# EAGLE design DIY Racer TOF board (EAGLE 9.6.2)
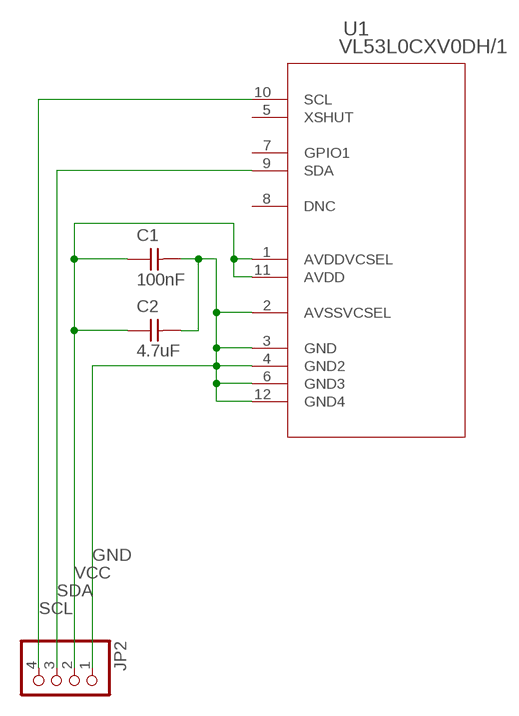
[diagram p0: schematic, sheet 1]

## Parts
C1  100nF  CAP_UNPOLARIZED  [C1206]
C2  4.7uF  CAP_UNPOLARIZED  [C1206]
JP2  PINHD-1X04_2.54-SMD  [1X04SMD]
U1  VL53L0CXV0DH/1  [LGA12_STM]

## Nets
GND: C1.2 C2.2 JP2.1 U1.2(AVSSVCSEL) U1.3(GND) U1.4(GND2) U1.6(GND3) U1.12(GND4)
SCL: JP2.4 U1.10(SCL)
SDA: JP2.3 U1.9(SDA)
VCC: C1.1 C2.1 JP2.2 U1.1(AVDDVCSEL) U1.11(AVDD)
Unconnected: U1.5(XSHUT) U1.7(GPIO1) U1.8(DNC)

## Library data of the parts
C1 C2 = fab:CAP_UNPOLARIZED
JP2 = pinhead-2:PINHD-1X04: PIN HEADER
U1 = VL53L0CXV0DH1:VL53L0CXV0DH/1; BUILT_BY: EMA_Jessica; COPYRIGHT: Copyright (C) 2018 Accelerated Designs. All rights reserved; MANUFACTURER_PART_NUMBER: VL53L0CXV0DH/1; SOURCELIBRARY: Update_to_database_2020-12-04; VENDOR: STMicroelectronics

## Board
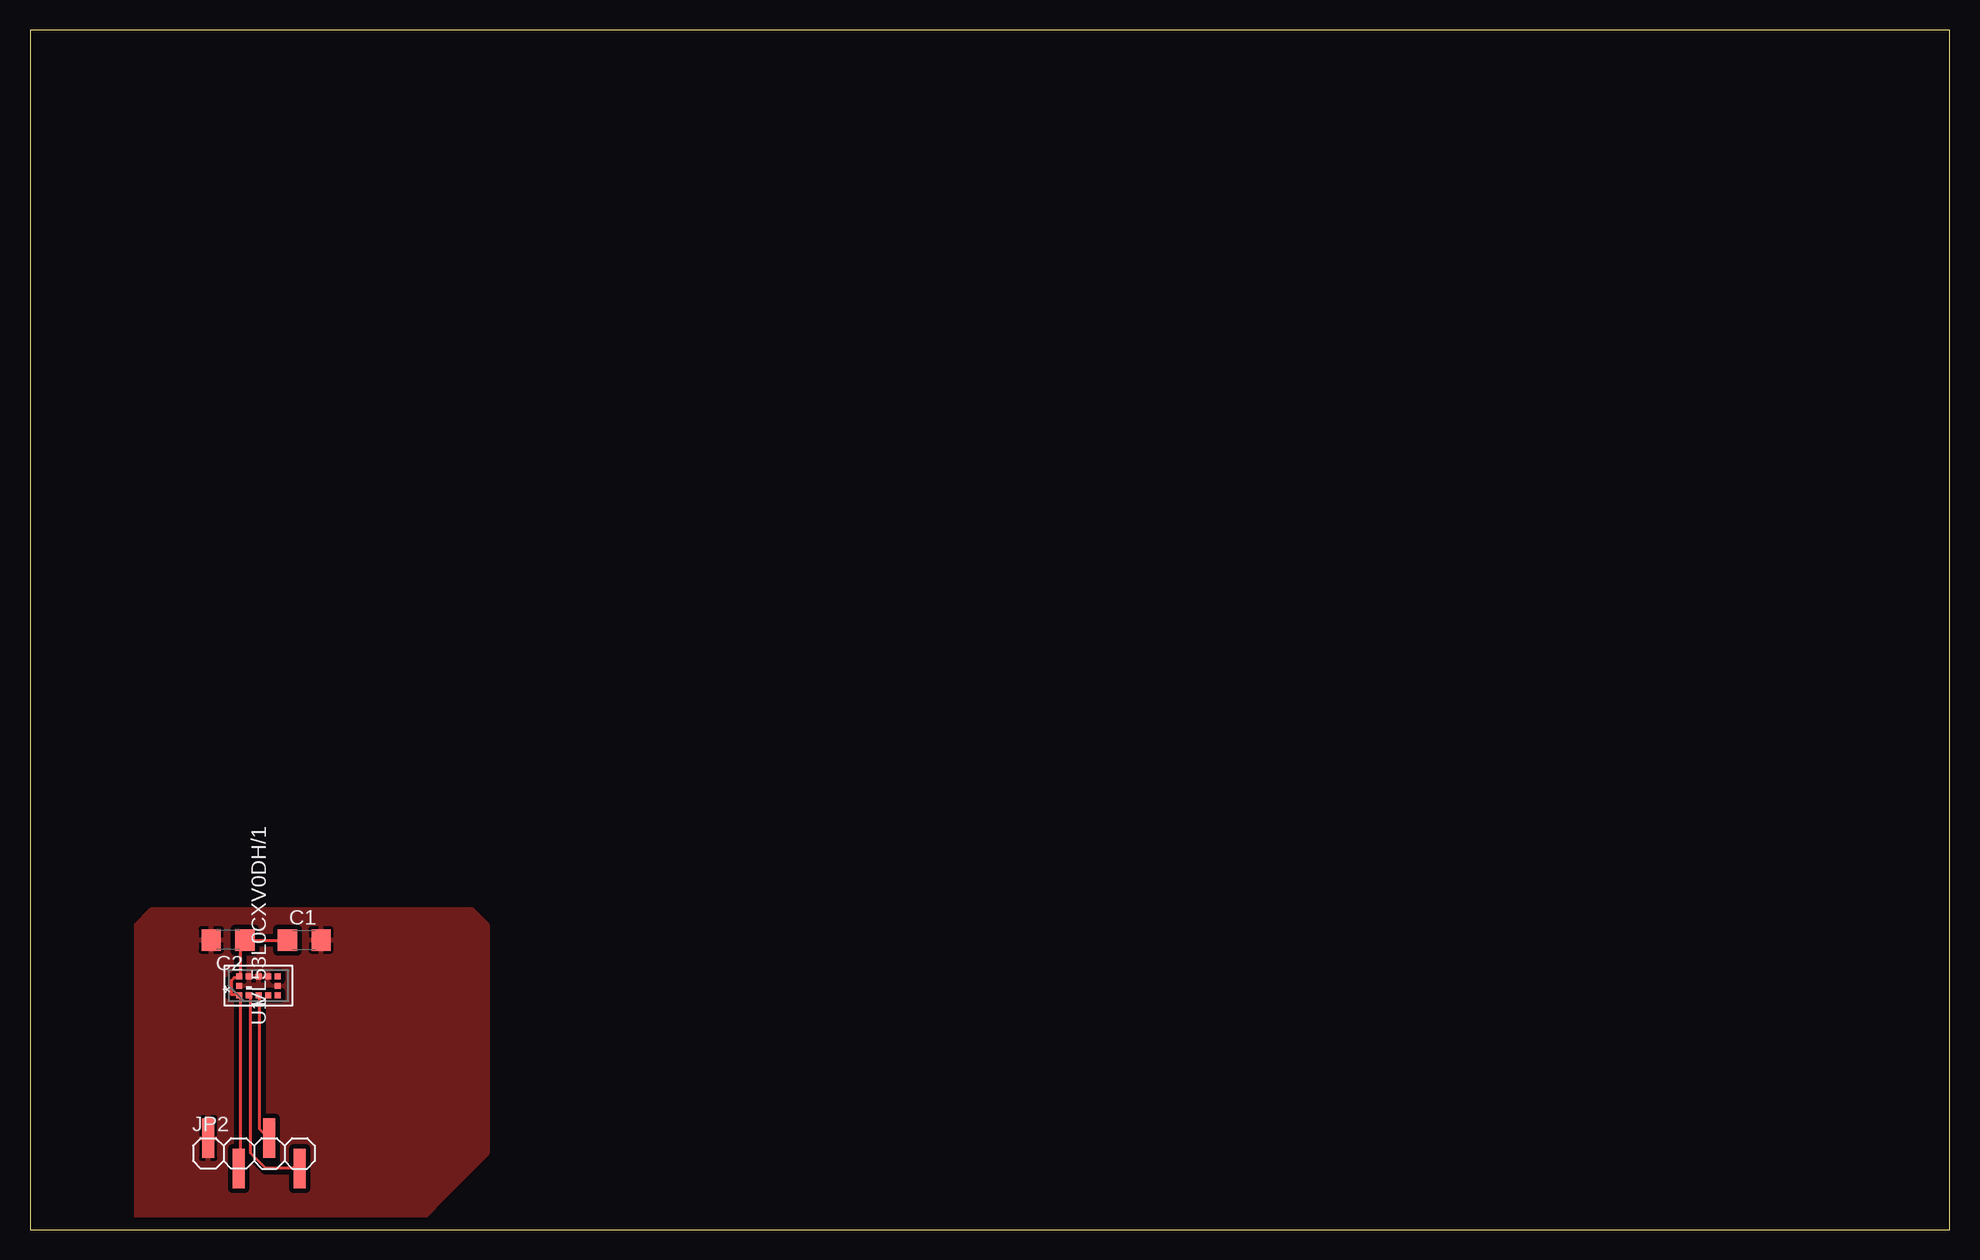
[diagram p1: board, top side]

Size 160 x 100 mm. Coordinates in mm from the lower left corner, seen from the top.
Outline: 0,0 160,0 160,100 0,100 0,0
Copper layers (1*16): Top 0.035mm / dielectric 1.5mm / Bottom 0.035mm
Design rules "default *": minimum track width 0.25mm, minimum drill 0.35mm, track to track 0.4mm, track to pad 0.25mm, pad to pad 0.25mm, via to via 0.4mm, smd to smd 0.25mm, copper to edge 40mil, drill to drill 6mil, minimum pad ring 10mil, minimum via ring 8mil, stop-mask expansion 4mil, vias tented up to drill 0mil, thermal gap 10mil

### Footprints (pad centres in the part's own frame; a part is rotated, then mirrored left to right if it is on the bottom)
C1206 = smd 1.6 x 1.8: 1 -1.4,0; 2 1.4,0
1X04SMD = smd 1.016 x 3.302: 1 -1.27,1.27; 2 1.27,-1.27; 3 3.81,1.27; 4 6.35,-1.27
LGA12_STM = smd 0.508 x 0.508: 1 0.8,1.6; 2 0.8,0.8; 3 0.8,0; 4 0.8,-0.8; 5 0.8,-1.6; 6 0,-1.6; 7 -0.8,-1.6; 8 -0.8,-0.8; 9 -0.8,0; 10 -0.8,0.8; 11 -0.8,1.6; 12 0,1.6

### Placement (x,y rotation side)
C1  22.86,24.13 0 top
C2  16.51,24.13 180 top
JP2  16.13,6.35 0 top
U1  19.05,20.32 90 top

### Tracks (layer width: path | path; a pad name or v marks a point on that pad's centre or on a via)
GND
  pour Top: 10.16,26.67 36.83,26.67 38.1,25.4 38.1,6.35 35.56,3.81 31.75,0 26.67,0 8.89,0 8.89,25.4
SCL
  Top 0.25: U1.10 18.25,19.5 18.38,19.38 18.38,6.38 19.62,5.12 22.38,5.12 JP2.4
SDA
  Top 0.25: U1.9 19.12,19.5 19.12,8.38 19.88,7.62 JP2.3
VCC
  Top 0.25: C1.1 21.38,24.12 18,24.12 C2.1 17.88,24.12 17.5,23.75 17.5,21.12 U1.1 17.38,21 17,21 16.75,20.75 16.75,19.62 17.38,19.62 U1.11 17.5,19.5 17.5,5.12 JP2.2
